(* Logix 5000 AddOnInstructionDefinition export AMCI_ANG1E_Run_Dwell_Move; software revision 20.03 *)

ADD_ON_INSTRUCTION AMCI_ANG1E_Run_Dwell_Move   (* revision 5.0, vendor AMCI, ExecuteEnableInFalse *)
// Revision note:
// Version 5.0 added the (hidden) ability to program the motor current and unlatched the error bit if the rung goes false.
VAR_INPUT
   Axis_Status_Bits : INT; {required}
   slot_axis_number : INT; {required}
   Assembed_Move_Dwell_Time : INT; {required}
   Type_0_for_standard_1_for_indexed : BOOL;
   motor_current : INT;
END_VAR
VAR_IN_OUT
   AMCI_ANG1E_output_data : INT[10]; {required}
END_VAR
VAR_OUTPUT
   EN : BOOL; {access Read Only, visible}
   ER : BOOL; {access Read Only, visible}
END_VAR
VAR
   command_data_block : INT[10];
        [0]   // Command Bits MSW
        [1]   // Command Bits LSW
        [2]   // Upper Target Position
        [3]   // Lower Target Position
        [4]   // Upper Programmed Speed
        [5]   // Lower Programmed Speed
   index : INT;
END_VAR

ROUTINE EnableInFalse   (* ladder *)
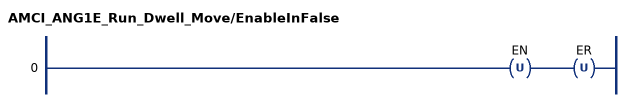
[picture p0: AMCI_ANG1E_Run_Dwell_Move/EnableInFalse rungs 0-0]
   0: OTU(EN)OTU(ER);
END_ROUTINE

ROUTINE Logic   (* ladder *)
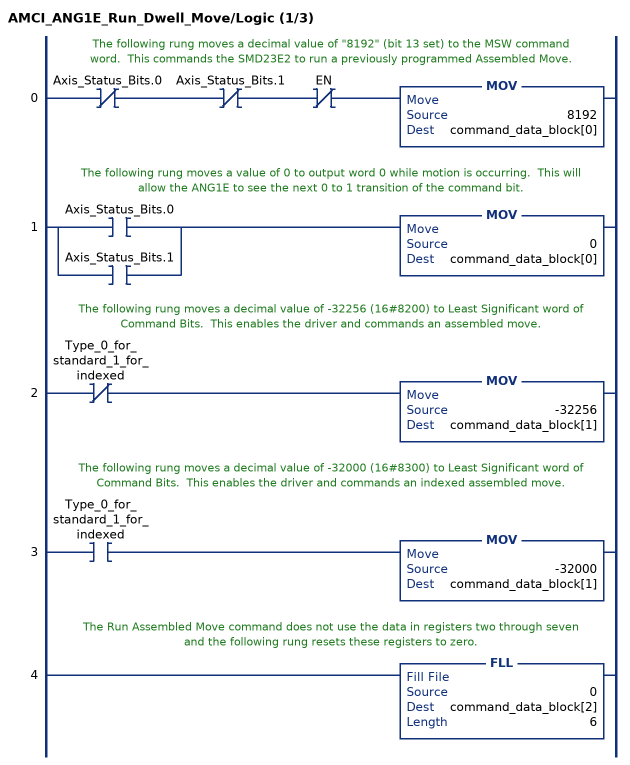
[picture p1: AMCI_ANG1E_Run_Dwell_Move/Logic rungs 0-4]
   // The following rung moves a decimal value of "8192" (bit 13 set) to the MSW command word.  This commands the SMD23E2 to run a previously programmed Assembled Move.
   0: XIO(Axis_Status_Bits.0)XIO(Axis_Status_Bits.1)XIO(EN)MOV(8192,command_data_block[0]);
   // The following rung moves a value of 0 to output word 0 while motion is occurring.  This will allow the ANG1E to see the next 0 to 1 transition of the command bit.
   1: [XIC(Axis_Status_Bits.0) ,XIC(Axis_Status_Bits.1) ]MOV(0,command_data_block[0]);
   // The following rung moves a decimal value of -32256 (16#8200) to Least Significant word of Command Bits.  This enables the driver and commands an assembled move.
   2: XIO(Type_0_for_standard_1_for_indexed)MOV(-32256,command_data_block[1]);
   // The following rung moves a decimal value of -32000 (16#8300) to Least Significant word of Command Bits.  This enables the driver and commands an indexed assembled move.
   3: XIC(Type_0_for_standard_1_for_indexed)MOV(-32000,command_data_block[1]);
   // The Run Assembled Move command does not use the data in registers two through seven and the following rung resets these registers to zero.
   4: FLL(0,command_data_block[2],6);
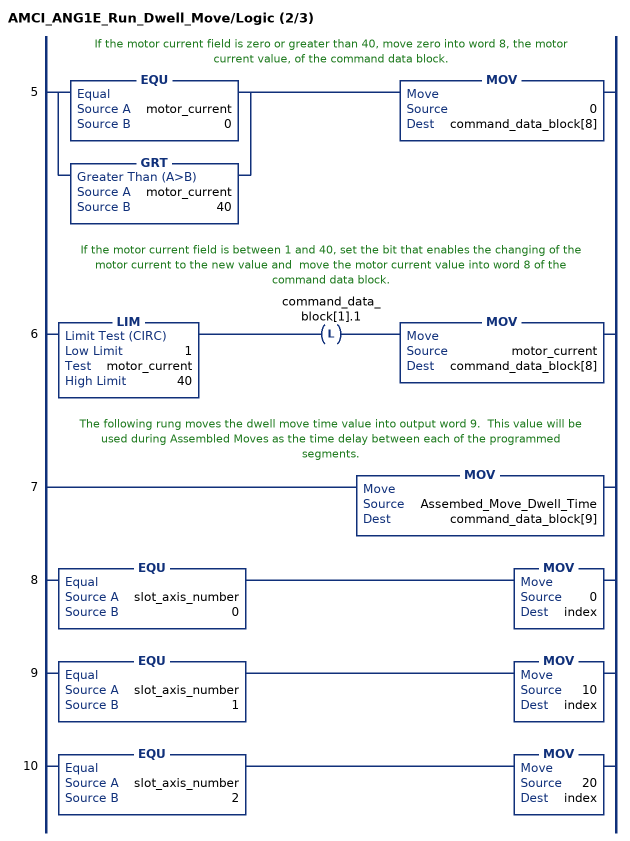
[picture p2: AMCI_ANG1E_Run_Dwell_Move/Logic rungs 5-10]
   // If the motor current field is zero or greater than 40, move zero into word 8, the motor current value, of the command data block.
   5: [EQU(motor_current,0) ,GRT(motor_current,40) ]MOV(0,command_data_block[8]);
   // If the motor current field is between 1 and 40, set the bit that enables the changing of the motor current to the new value and  move the motor current value into word 8 of the command data block.
   6: LIM(1,motor_current,40)OTL(command_data_block[1].1)MOV(motor_current,command_data_block[8]);
   // The following rung moves the dwell move time value into output word 9.  This value will be used during Assembled Moves as the time delay between each of the programmed segments.
   7: MOV(Assembed_Move_Dwell_Time,command_data_block[9]);
   8: EQU(slot_axis_number,0)MOV(0,index);
   9: EQU(slot_axis_number,1)MOV(10,index);
   10: EQU(slot_axis_number,2)MOV(20,index);
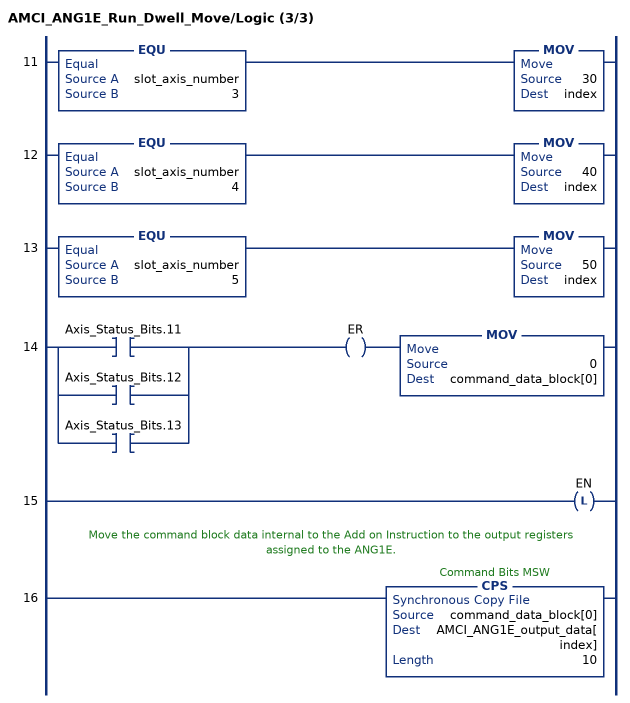
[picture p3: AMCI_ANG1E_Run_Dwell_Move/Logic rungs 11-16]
   11: EQU(slot_axis_number,3)MOV(30,index);
   12: EQU(slot_axis_number,4)MOV(40,index);
   13: EQU(slot_axis_number,5)MOV(50,index);
   14: [XIC(Axis_Status_Bits.11) ,XIC(Axis_Status_Bits.12) ,XIC(Axis_Status_Bits.13) ]OTE(ER)MOV(0,command_data_block[0]);
   15: OTL(EN);
   // Move the command block data internal to the Add on Instruction to the output registers assigned to the ANG1E.
   16: CPS(command_data_block[0],AMCI_ANG1E_output_data[index],10);
END_ROUTINE
END_ADD_ON_INSTRUCTION
